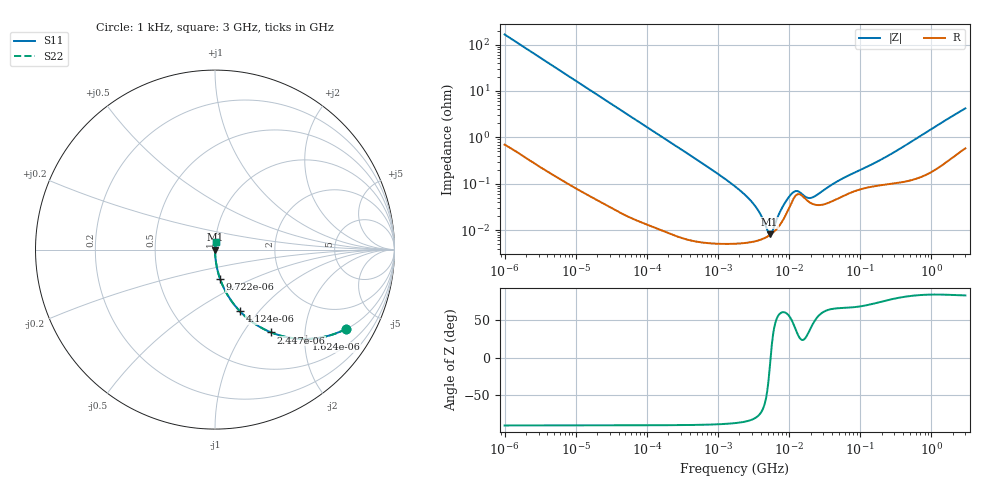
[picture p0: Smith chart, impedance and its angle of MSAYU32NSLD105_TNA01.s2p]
! MSAYU32NSLD105_TNA01  S-PARAMETER MODEL  ( Standard Model )
! Model Generated by TAIYO YUDEN Corporation (http://www.ty-top.com)
! Version 1.0
! TAIYO YUDEN Control No. 220601
! Copyright(c) 2012 TAIYO YUDEN CO.,LTD. All Rights Reserved.
! Product Description (link to TY-COMPAS)
! https://ds.yuden.co.jp/TYCOMPAS/or/detail?pn=MSAYU32NSLD105KTNA01&u=M
! Products Name : Multilayer Ceramic Capacitors
! Characteristics :
!  Capacitance : 1 [uF] , Rated Voltage : 50 [V] , TCC : X5R
!  Case Size : 3.2 x 2.5 / 0.126 x 0.098 [mm/inch] , Thickness : 1.9 / 0.075 [mm/inch]
!  (Conditions: Temperature = 25 [degC] , DC Bias Voltage = 0 [V])
! External Node Assignments :
!  1  o---| |---o  2
! GND o---------o GND
! Frequency Range : 1kHz  -  3GHz  [ 401 STEP ]
# MHZ S RI R 50
! Freq[MHz].  S11 Real  S11 Imag  S21 Real  S21 Imag  S12 Real  S12 Imag  S22 Real  S22 Imag
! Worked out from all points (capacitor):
!   401 points, 1 kHz to 3 GHz, reference 50 ohm
!   read as one part in series: C = 966 nF near 1.077 kHz
!   lowest |Z| = 8.1 mohm at 5.301 MHz (marker M1)
!   series resonance near 5.486 MHz, so ESL is about 870 pH
!   S11 on the Smith chart (normalised r, x): 1 kHz: 1.01, -3.29; 1.624 kHz: 1.01, -2.03; 2.447 kHz: 1.01, -1.35; 4.124 kHz: 1.00, -0.80; 9.722 kHz: 1.00, -0.34; 3 GHz: 1.01, +0.08
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0.001  0.7295 -0.4421  0.2705 0.4421  0.2705 0.4421  0.7295 -0.4421
0.001624  0.5075 -0.4978  0.4925 0.4978  0.4925 0.4978  0.5075 -0.4978
0.002447  0.3134 -0.4617  0.6866 0.4617  0.6866 0.4617  0.3134 -0.4617
0.004124  0.1394 -0.3442  0.8606 0.3442  0.8606 0.3442  0.1394 -0.3442
0.009722  0.029 -0.1653  0.971 0.1653  0.971 0.1653  0.029 -0.1653
0.01216  0.0189 -0.1336  0.9811 0.1336  0.9811 0.1336  0.0189 -0.1336
0.033275  0.00278 -0.0498  0.9972 0.0498  0.9972 0.0498  0.00278 -0.0498
0.147855  0.000232 -0.0113  0.9998 0.0113  0.9998 0.0113  0.000232 -0.0113
1.732051  5.18e-05 -0.000878  0.9999 0.000878  0.9999 0.000878  5.18e-05 -0.000878
3.14518  5.67e-05 -0.000366  0.9999 0.000366  0.9999 0.000366  5.67e-05 -0.000366
3.93371  6.22e-05 -0.000214  0.9999 0.000214  0.9999 0.000214  6.22e-05 -0.000214
4.739869  7.03e-05 -9.43e-05  0.9999 9.43e-05  0.9999 9.43e-05  7.03e-05 -9.43e-05
5.30084  7.78e-05 -2.23e-05  0.9999 2.23e-05  0.9999 2.23e-05  7.78e-05 -2.23e-05
5.928204  8.88e-05 5.12e-05  0.9999 -5.12e-05  0.9999 -5.12e-05  8.88e-05 5.12e-05
8.291982  0.000171 0.000295  0.9998 -0.000295  0.9998 -0.000295  0.000171 0.000295
11.1738  0.000437 0.000466  0.9996 -0.000466  0.9996 -0.000466  0.000437 0.000466
12.97096  0.000589 0.000371  0.9994 -0.000371  0.9994 -0.000371  0.000589 0.000371
17.47891  0.000452 0.000238  0.9995 -0.000238  0.9995 -0.000238  0.000452 0.000238
21.06097  0.000371 0.000343  0.9996 -0.000343  0.9996 -0.000343  0.000371 0.000343
51.53541  0.000505 0.0011  0.9995 -0.0011  0.9995 -0.0011  0.000505 0.0011
256.0921  0.000999 0.00405  0.999 -0.00405  0.999 -0.00405  0.000999 0.00405
3000  0.00747 0.0412  0.9925 -0.0412  0.9925 -0.0412  0.00747 0.0412
